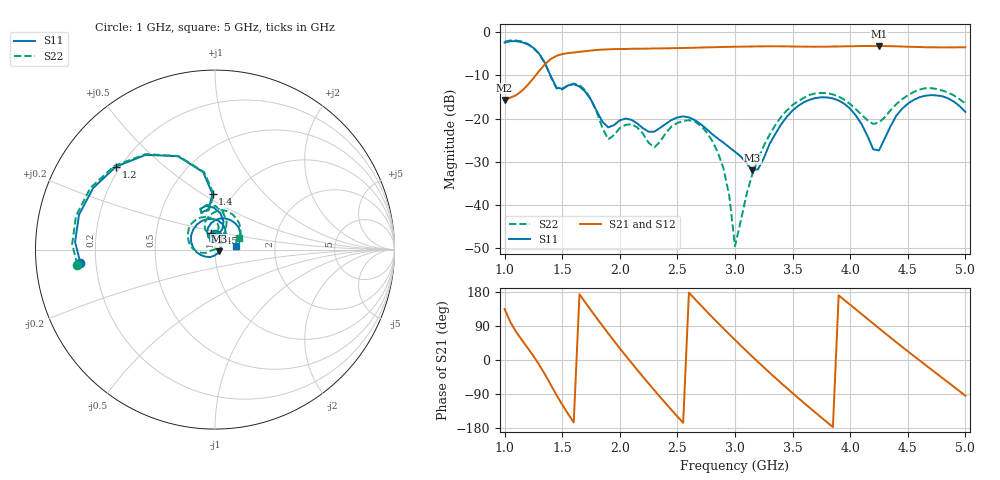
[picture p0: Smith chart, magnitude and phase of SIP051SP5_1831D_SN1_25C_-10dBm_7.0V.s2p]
# GHz  S  dB  R  50
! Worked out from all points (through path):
!   81 points, 1 GHz to 5 GHz, reference 50 ohm
!   highest |S21| = -3.24 dB at 4.25 GHz (marker M1); lowest = -15.7 dB at 1 GHz (marker M2)
!   lowest |S11| = -31.9 dB at 3.15 GHz (marker M3), VSWR 1.05, Z = 52.4 - j1.07 ohm
!   |S11| at or under -10 dB: 1.397 GHz to end of sweep
!   |S22| runs from -49.5 to -2.0 dB; largest |S21 - S12| = 0.0035
!   S11 on the Smith chart (normalised r, x): 1 GHz: 0.14, -0.05; 1.2 GHz: 0.18, +0.35; 1.4 GHz: 0.81, +0.55; 2.45 GHz: 0.94, +0.18; 5 GHz: 1.27, +0.05
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1  -2.46 -174.4  -15.74 134.8  -15.73 134.9  -2.25 -173.7
1.2  -2.85 140.0  -12.28 31.9  -12.27 32.0  -2.74 140.2
1.4  -10.19 92.4  -6.28 -64.9  -6.29 -64.7  -10.25 91.3
1.5  -13.13 110.1  -5.12 -117.7  -5.11 -117.6  -13.29 110.5
1.7  -13.79 81.4  -4.45 152.1  -4.45 152.2  -13.49 77.5
1.85  -20.81 76.8  -4.08 90.0  -4.08 90.2  -22.27 63.6
2.05  -20.02 99.7  -3.94 11.8  -3.94 11.8  -21.48 101.1
2.2  -22.22 90.8  -3.87 -43.9  -3.86 -43.9  -23.46 85.0
2.35  -22.16 108.0  -3.81 -97.5  -3.81 -97.5  -25.35 119.2
2.45  -20.33 103.7  -3.76 -132.2  -3.77 -132.1  -21.82 118.8
2.6  -19.75 79.1  -3.68 177.8  -3.68 177.9  -20.39 87.9
2.8  -23.57 53.3  -3.54 113.8  -3.54 113.8  -25.07 49.1
2.9  -25.57 45.0  -3.48 83.0  -3.47 83.1  -31.51 38.8
3  -27.68 35.2  -3.42 53.0  -3.41 52.9  -49.49 60.4
3.15  -31.93 -23.7  -3.36 9.0  -3.36 9.2  -32.91 -166.3
3.45  -19.60 -172.9  -3.34 -74.3  -3.35 -74.2  -18.11 177.4
3.7  -15.27 125.8  -3.41 -139.3  -3.41 -139.2  -14.19 132.2
3.95  -16.62 73.0  -3.33 158.1  -3.34 158.2  -15.69 91.1
4.25  -27.38 97.0  -3.24 83.7  -3.25 83.8  -20.94 107.7
4.35  -21.80 117.3  -3.30 59.2  -3.29 59.3  -18.11 116.0
4.65  -14.76 71.5  -3.54 -12.3  -3.52 -12.4  -13.01 79.9
5  -18.47 9.7  -3.54 -94.4  -3.54 -94.2  -16.56 25.6
